| IBIS file MPC8308_ibis.ibs generated by Viper version: 2008.08.r27
[IBIS Ver]   4.2
[Comment Char]   |_char
[File Name]   mpc8308_ibis_19072011.ibs
[File Rev]   B
[Date]   Mon Nov 2 12:15:30 2009
[Source]   Generated using: Viper
[Notes]   Updated pulldown data  for ddr1_type_drv_io model.
[Disclaimer]
[Copyright]   Copyright (C) 1998 - 2004 Freescale Semiconductor Israel Ltd.
|   MPC8308
[Component]   MPC8308
[Manufacturer]   FREESCALE
[Package]
| variable   typ   min   max
R_pkg   326.285m   89.855m   584.065m
L_pkg   4.52nH   1.32nH   7.74nH
C_pkg   1.88pF   0.974pF   6.09pF
[Pin] signal_name   model_name   R_pin   L_pin   C_pin
A1   GVDD   POWER   2.35E-01  3.44E-09  4.55E-12
A10   XPADVSS   GND   NA   NA   NA
A11   SD_IMP_CAL_TX   tx_pzctl   4.46E-01  5.33E-09  9.95E-13
A12   XCOREVSS   GND   NA   NA   NA
A13   RXA   ptrmr100_cm   4.10E-01  4.92E-09  1.01E-12
A14   XCOREVDD   POWER   1.42E-01  2.40E-09  3.60E-12
A15   SD_IMP_CAL_RX   rx_pzctl   5.04E-01  6.02E-09  1.03E-12
A16   NVDDB   POWER   3.74E-01  5.65E-09  2.94E-12
A17   IRQ_B0   Progbuffer1   4.01E-01  5.91E-09  1.08E-12
A18   IRQ_B3   Progbuffer1   4.06E-01  5.79E-09  1.14E-12
A19   NVDDB   POWER   3.74E-01  5.65E-09  2.94E-12
A2   VSS   GND   NA   NA   NA
A20   TSEC1_MDC   Progbuffer1   4.23E-01  6.17E-09  1.26E-12
A21   VSS   GND   NA   NA   NA
A22   TSEC1_RX_CLK   Progbuffer1   3.77E-01  6.03E-09  1.75E-12
A23   NVDDC   POWER   4.46E-01  5.97E-09  4.02E-12
A3   MEMC_MCK0   Progbuffer2   4.19E-01  6.14E-09  1.33E-12
A4   MEMC_MCK_B0   Progbuffer2   4.10E-01  6.18E-09  1.30E-12
A5   MEMC_MODT0   Progbuffer2   4.18E-01  6.07E-09  1.18E-12
A6   GVDD   POWER   2.35E-01  3.44E-09  4.55E-12
A7   SD_CD_B   Progbuffer1   3.90E-01  5.44E-09  1.24E-12
A8   SD_DAT2   Progbuffer1   3.81E-01  5.40E-09  1.20E-12
A9   IIC_SCL1   Progbuffer1   4.00E-01  5.74E-09  1.05E-12
AA1   MEMC_MDQ5   Progbuffer2   4.30E-01  6.08E-09  1.53E-12
AA10  LGPL1   Progbuffer1   3.51E-01  4.78E-09  1.18E-12
AA11  NVDDK   POWER   1.50E-01  2.43E-09  6.05E-12
AA12  LCS_B2   Progbuffer1   3.61E-01  4.89E-09  1.29E-12
AA13  LCS_B0   Progbuffer1   3.61E-01  4.88E-09  1.29E-12
AA14  LA20   Progbuffer1   3.52E-01  4.95E-09  1.32E-12
AA15  LA12   Progbuffer1   3.58E-01  4.62E-09  1.34E-12
AA16  LA7   Progbuffer1   3.62E-01  5.03E-09  1.48E-12
AA17  LA5   Progbuffer1   3.75E-01  5.29E-09  1.43E-12
AA18  LA4   Progbuffer1   3.88E-01  5.52E-09  1.46E-12
AA19  LD14   Progbuffer1   3.96E-01  5.64E-09  1.52E-12
AA2   MEMC_MDQ4   Progbuffer2   4.01E-01  5.83E-09  1.64E-12
AA20  LD9   Progbuffer1   4.03E-01  5.73E-09  1.47E-12
AA21  LD4   Progbuffer1   4.06E-01  5.85E-09  1.62E-12
AA22  STBY_VBAT   POWER   2.25E-01  3.87E-09  1.83E-12
AA23  RTC_PIT_CLOCK   Progbuffer1   4.29E-01  6.45E-09  1.34E-12
AA3   MEMC_MDQ3   Progbuffer2   3.92E-01  5.55E-09  1.55E-12
AA4   VSS   GND   NA   NA   NA
AA5   SPICLK   Progbuffer1   3.43E-01  4.74E-09  1.42E-12
AA6   TMS   Progbuffer1   3.67E-01  5.05E-09  1.34E-12
AA7   QUIESCE_B   Progbuffer1   3.63E-01  4.98E-09  1.27E-12
AA8   PORESET_B   Progbuffer1   3.50E-01  4.77E-09  1.23E-12
AA9   HRESET_B   Progbuffer1   3.53E-01  4.75E-09  1.26E-12
AB1   VSS   GND   NA   NA   NA
AB10  LGPL2   Progbuffer1   3.80E-01  4.89E-09  1.17E-12
AB11  LWE_B0   Progbuffer1   3.46E-01  4.72E-09  1.20E-12
AB12  VSS   GND   NA   NA   NA
AB13  LCS_B1   Progbuffer1   3.82E-01  5.40E-09  1.38E-12
AB14  LA21   Progbuffer1   3.71E-01  5.30E-09  1.27E-12
AB15  LA19   Progbuffer1   3.80E-01  5.48E-09  1.33E-12
AB16  NVDDK   POWER   1.50E-01  2.43E-09  6.05E-12
AB17  LA11   Progbuffer1   3.92E-01  5.66E-09  1.37E-12
AB18  LA8   Progbuffer1   4.06E-01  5.89E-09  1.49E-12
AB19  VSS   GND   NA   NA   NA
AB2   MEMC_MDM0   Progbuffer2   4.21E-01  6.20E-09  1.52E-12
AB20  LD12   Progbuffer1   4.21E-01  6.12E-09  1.50E-12
AB21  LD7   Progbuffer1   4.37E-01  6.14E-09  1.54E-12
AB22  NVDDK   POWER   1.50E-01  2.43E-09  6.05E-12
AB23  NVDDJ   POWER   3.92E-01  5.82E-09  1.51E-12
AB3   MEMC_MDQ2   Progbuffer2   3.99E-01  5.92E-09  1.57E-12
AB4   SPISEL   Progbuffer1   3.73E-01  5.49E-09  1.44E-12
AB5   SPIMOSI   Progbuffer1   3.84E-01  5.45E-09  1.34E-12
AB6   VSS   GND   NA   NA   NA
AB7   SRESET_B   Progbuffer1   3.87E-01  5.24E-09  1.25E-12
AB8   NVDDP   POWER   1.50E-01  2.43E-09  6.05E-12
AB9   LGPL4   Progbuffer1   3.69E-01  5.11E-09  1.22E-12
AC1   GVDD   POWER   2.35E-01  3.44E-09  4.55E-12
AC10  LGPL3   Progbuffer1   3.90E-01  5.49E-09  1.04E-12
AC11  LWE_B1   Progbuffer1   3.70E-01  5.17E-09  1.22E-12
AC12  LCLK0   Progbuffer1   3.22E-01  4.34E-09  1.35E-12
AC13  NVDDK   POWER   1.50E-01  2.43E-09  6.05E-12
AC14  LA25   Progbuffer1   4.15E-01  5.88E-09  1.18E-12
AC15  LA15   Progbuffer1   3.91E-01  5.37E-09  1.22E-12
AC16  LA13   Progbuffer1   4.12E-01  5.89E-09  1.18E-12
AC17  LD15   Progbuffer1   3.90E-01  5.61E-09  1.46E-12
AC18  LA9   Progbuffer1   4.29E-01  6.14E-09  1.25E-12
AC19  LA6   Progbuffer1   4.31E-01  6.45E-09  1.27E-12
AC2   VSS   GND   NA   NA   NA
AC20  LA0   Progbuffer1   4.38E-01  6.54E-09  1.31E-12
AC21  LD11   Progbuffer1   4.44E-01  6.62E-09  1.33E-12
AC22  LD5   Progbuffer1   4.50E-01  6.71E-09  1.37E-12
AC23  VSS   GND   NA   NA   NA
AC3   MEMC_MDQS0   Progbuffer2   3.56E-01  5.44E-09  1.71E-12
AC4   NVDDP   POWER   1.50E-01  2.43E-09  6.05E-12
AC5   TDO   Progbuffer1   4.17E-01  5.78E-09  1.15E-12
AC6   TEST_MODE   Progbuffer1   3.98E-01  5.75E-09  1.42E-12
AC7   THERM0   Progbuffer1   3.98E-01  5.69E-09  1.11E-12
AC8   SYS_CLK_IN   Progbuffer1   3.33E-01  4.31E-09  1.32E-12
AC9   VSS   GND   NA   NA   NA
B1   VSS   GND   NA   NA   NA
B10   NVDDA   POWER   5.84E-01  7.74E-09  2.08E-12
B12   XCOREVDD   POWER   1.42E-01  2.40E-09  3.60E-12
B13   RXA_B   ptrmr100_cm   4.19E-01  5.41E-09  9.74E-13
B14   XCOREVSS   GND   NA   NA   NA
B15   XPADVSS   GND   NA   NA   NA
B17   IRQ_B2   Progbuffer1   3.79E-01  5.27E-09  1.28E-12
B18   UART_SIN1   Progbuffer1   3.86E-01  5.42E-09  1.29E-12
B19   VSS   GND   NA   NA   NA
B2   MEMC_MBA1   Progbuffer2   4.31E-01  6.26E-09  1.61E-12
B20   TSEC1_COL   Progbuffer1   4.00E-01  5.55E-09  1.44E-12
B21   TSEC1_CRS   Progbuffer1   4.09E-01  6.01E-09  1.66E-12
B22   NVDDC   POWER   4.46E-01  5.97E-09  4.02E-12
B23   VSS   GND   NA   NA   NA
B3   GVDD   POWER   2.35E-01  3.44E-09  4.55E-12
B4   MEMC_MRAS_B   Progbuffer2   4.12E-01  5.84E-09  1.29E-12
B5   MEMC_MODT1   Progbuffer2   3.96E-01  5.64E-09  1.36E-12
B6   MEMC_MCS_B0   Progbuffer2   3.95E-01  5.51E-09  1.29E-12
B7   NVDDA   POWER   5.84E-01  7.74E-09  2.08E-12
B8   SD_DAT1   Progbuffer1   3.54E-01  4.87E-09  1.23E-12
B9   SD_DAT3   Progbuffer1   3.76E-01  5.12E-09  1.23E-12
C1   MEMC_MA10   Progbuffer2   4.47E-01  6.37E-09  1.34E-12
C10   IIC_SCL2   Progbuffer1   3.68E-01  4.89E-09  1.03E-12
C11   XCOREVSS   GND   NA   NA   NA
C12   SD_REF_CLK_B   ptrmr100_cm   3.86E-01  3.95E-09  1.24E-12
C13   XCOREVDD   POWER   1.42E-01  2.40E-09  3.60E-12
C14   TXA   tx_select   3.56E-01  4.78E-09  1.04E-12
C15   TXA_B   tx_select   3.89E-01  4.01E-09  1.07E-12
C16   VSS   GND   NA   NA   NA
C17   UART_SOUT1   Progbuffer1   3.63E-01  4.99E-09  1.33E-12
C18   NVDDB   POWER   3.74E-01  5.65E-09  2.94E-12
C19   TSEC1_MDIO   Progbuffer1   3.76E-01  5.23E-09  1.38E-12
C2   MEMC_MA0   Progbuffer2   4.29E-01  5.96E-09  1.61E-12
C20   TSEC1_RXD1   Progbuffer1   3.87E-01  5.59E-09  1.64E-12
C21   TSEC1_RXD2   Progbuffer1   3.90E-01  5.55E-09  1.46E-12
C22   TSEC1_RXD3   Progbuffer1   4.07E-01  5.90E-09  1.43E-12
C23   TSEC1_RX_ER   Progbuffer1   4.23E-01  6.20E-09  1.29E-12
C3   MEMC_MBA0   Progbuffer2   4.01E-01  5.71E-09  1.56E-12
C4   VSS   GND   NA   NA   NA
C5   MEMC_MCAS_B   Progbuffer2   3.68E-01  5.10E-09  1.38E-12
C6   MEMC_MCS_B1   Progbuffer2   3.77E-01  4.73E-09  1.31E-12
C7   NVDDA   POWER   5.84E-01  7.74E-09  2.08E-12
C8   SD_DAT0   Progbuffer1   3.50E-01  4.30E-09  1.21E-12
C9   IIC_SDA1   Progbuffer1   3.34E-01  4.26E-09  1.26E-12
D1   GVDD   POWER   2.35E-01  3.44E-09  4.55E-12
D10   IIC_SDA2   Progbuffer1   2.93E-01  3.86E-09  1.41E-12
D11   XCOREVSS   GND   NA   NA   NA
D12   SD_REF_CLK   ptrmr100_cm   3.46E-01  4.30E-09  1.23E-12
D13   XCOREVSS   GND   NA   NA   NA
D14   XPADVSS   GND   NA   NA   NA
D15   XPADVDD   POWER   2.04E-01  2.96E-09  2.44E-12
D17   UART_SOUT2   Progbuffer1   3.57E-01  4.45E-09  1.34E-12
D18   UART_SIN2   Progbuffer1   3.57E-01  4.77E-09  1.37E-12
D19   VSS   GND   NA   NA   NA
D2   MEMC_MA1   Progbuffer2   4.13E-01  5.94E-09  1.47E-12
D20   TSEC1_RXD0   Progbuffer1   3.63E-01  5.08E-09  1.53E-12
D21   TSEC1_RX_DV   Progbuffer1   3.82E-01  5.44E-09  1.42E-12
D22   TSEC1_TXD0   Progbuffer1   4.01E-01  5.76E-09  1.39E-12
D23   NVDDC   POWER   4.46E-01  5.97E-09  4.02E-12
D3   MEMC_MA2   Progbuffer2   4.15E-01  5.34E-09  1.54E-12
D4   MEMC_MA3   Progbuffer2   3.66E-01  5.13E-09  1.56E-12
D5   MEMC_MWE_B   Progbuffer2   3.76E-01  4.73E-09  1.54E-12
D6   VSS   GND   NA   NA   NA
D7   SD_CLK   Progbuffer1   3.49E-01  4.40E-09  1.14E-12
D8   SD_WP   Progbuffer1   3.31E-01  4.41E-09  1.40E-12
D9   NVDDA   POWER   5.84E-01  7.74E-09  2.08E-12
E1   MEMC_MA7   Progbuffer2   4.18E-01  6.10E-09  1.20E-12
E2   MEMC_MA6   Progbuffer2   3.99E-01  5.66E-09  1.38E-12
E20   NVDDC   POWER   4.46E-01  5.97E-09  4.02E-12
E21   TSEC1_TXD1   Progbuffer1   3.76E-01  5.28E-09  1.33E-12
E22   TSEC1_TX_ER   Progbuffer1   3.94E-01  5.60E-09  1.35E-12
E23   TSEC1_TX_CLK   Progbuffer1   3.45E-01  4.53E-09  1.55E-12
E3   VSS   GND   NA   NA   NA
E4   MEMC_MA4   Progbuffer2   3.67E-01  5.06E-09  1.48E-12
F1   GVDD   POWER   2.35E-01  3.44E-09  4.55E-12
F10   XPADVDD   POWER   2.04E-01  2.96E-09  2.44E-12
F11   SD_PLL_TPA_ANA   pad_ae   3.68E-01  3.88E-09  1.30E-12
F12   SDAVSS_0   GND   NA   NA   NA
F13   SD_PLL_TPD   pouv_out   3.43E-01  4.45E-09  1.40E-12
F14   XPADVDD   POWER   2.04E-01  2.96E-09  2.44E-12
F15   VSS   GND   NA   NA   NA
F16   IRQ_B1   Progbuffer1   3.44E-01  4.62E-09  1.46E-12
F17   VSS   GND   NA   NA   NA
F18   TSEC1_GTX_CLK   Progbuffer1   2.67E-01  3.07E-09  1.52E-12
F2   MEMC_MA8   Progbuffer2   3.90E-01  5.56E-09  1.40E-12
F20   TSEC1_TX_EN   Progbuffer1   3.51E-01  4.76E-09  1.34E-12
F21   TSEC1_TXD2   Progbuffer1   3.75E-01  5.23E-09  1.32E-12
F22   TSEC1_TXD3   Progbuffer1   3.90E-01  5.49E-09  1.33E-12
F23   VSS   GND   NA   NA   NA
F3   MEMC_MA9   Progbuffer2   3.75E-01  5.12E-09  1.37E-12
F4   MEMC_MA5   Progbuffer2   3.56E-01  4.86E-09  1.39E-12
F6   GVDD   POWER   2.35E-01  3.44E-09  4.55E-12
F7   MEMC_MA11   Progbuffer2   3.28E-01  4.28E-09  1.43E-12
F8   VSS   GND   NA   NA   NA
F9   NVDDA   POWER   5.84E-01  7.74E-09  2.08E-12
G1   MEMC_MCK2   Progbuffer2   3.89E-01  5.64E-09  1.21E-12
G10   VSS   GND   NA   NA   NA
G11   XCOREVSS   GND   NA   NA   NA
G12   SDAVDD_0   POWER   3.65E-01  4.85E-09  1.49E-12
G13   XPADVSS   GND   NA   NA   NA
G14   XPADVSS   GND   NA   NA   NA
G15   VSS   GND   NA   NA   NA
G16   VSS   GND   NA   NA   NA
G17   VSS   GND   NA   NA   NA
G18   NVDDC   POWER   4.46E-01  5.97E-09  4.02E-12
G2   MEMC_MA12   Progbuffer2   3.87E-01  5.48E-09  1.39E-12
G20   VSS   GND   NA   NA   NA
G21   GPIO_0   Progbuffer1   3.65E-01  5.05E-09  1.27E-12
G22   NVDDF   POWER   2.32E-01  3.22E-09  3.90E-12
G23   GPIO_3   Progbuffer1   3.47E-01  4.68E-09  1.22E-12
G3   MEMC_MA13   Progbuffer2   3.69E-01  5.12E-09  1.42E-12
G4   GVDD   POWER   2.35E-01  3.44E-09  4.55E-12
G6   MEMC_MVREF   Progbuffer2   1.31E-01  1.93E-09  1.74E-12
G7   VSS   GND   NA   NA   NA
G8   VSS   GND   NA   NA   NA
G9   SD_CMD   Progbuffer1   3.55E-01  4.81E-09  1.52E-12
H1   MEMC_MCK_B2   Progbuffer2   3.89E-01  5.72E-09  1.18E-12
H10   VDD   POWER   8.99E-02  1.32E-09  2.08E-12
H11   XCOREVSS   GND   NA   NA   NA
H12   XPADVSS   GND   NA   NA   NA
H13   XCOREVSS   GND   NA   NA   NA
H14   VDD   POWER   8.99E-02  1.32E-09  2.08E-12
H15   VDD   POWER   8.99E-02  1.32E-09  2.08E-12
H16   VDD   POWER   8.99E-02  1.32E-09  2.08E-12
H17   VSS   GND   NA   NA   NA
H18   GPIO_2   Progbuffer1   2.38E-01  2.74E-09  1.52E-12
H2   VSS   GND   NA   NA   NA
H20   GPIO_8   Progbuffer1   3.39E-01  4.55E-09  1.29E-12
H21   GPIO_7   Progbuffer1   3.59E-01  4.93E-09  1.30E-12
H22   GPIO_6   Progbuffer1   3.74E-01  5.21E-09  1.26E-12
H23   VSS   GND   NA   NA   NA
H3   MEMC_MCKE   Progbuffer2   3.38E-01  4.53E-09  1.24E-12
H4   MEMC_MBA2   Progbuffer2   3.32E-01  4.37E-09  1.56E-12
H6   VSS   GND   NA   NA   NA
H7   VSS   GND   NA   NA   NA
H8   VDD   POWER   8.99E-02  1.32E-09  2.08E-12
H9   VDD   POWER   8.99E-02  1.32E-09  2.08E-12
J1   GVDD   POWER   2.35E-01  3.44E-09  4.55E-12
J10   VSS   GND   NA   NA   NA
J11   VSS   GND   NA   NA   NA
J12   VSS   GND   NA   NA   NA
J13   VSS   GND   NA   NA   NA
J14   VSS   GND   NA   NA   NA
J15   VSS   GND   NA   NA   NA
J16   VDD   POWER   8.99E-02  1.32E-09  2.08E-12
J17   GPIO_14   Progbuffer1   3.60E-01  4.91E-09  1.59E-12
J18   GPIO_4   Progbuffer1   3.36E-01  4.48E-09  1.35E-12
J2   MEMC_MECC4   Progbuffer2   3.71E-01  5.16E-09  1.26E-12
J20   GPIO_5   Progbuffer1   3.34E-01  4.50E-09  1.23E-12
J21   GPIO_9   Progbuffer1   3.53E-01  4.85E-09  1.25E-12
J22   NVDDF   POWER   2.32E-01  3.22E-09  3.90E-12
J23   GPIO_10   Progbuffer1   3.40E-01  4.46E-09  1.13E-12
J3   MEMC_MECC6   Progbuffer2   3.57E-01  4.87E-09  1.27E-12
J4   GVDD   POWER   2.35E-01  3.44E-09  4.55E-12
J6   MEMC_MECC7   Progbuffer2   3.41E-01  4.39E-09  1.32E-12
J7   VSS   GND   NA   NA   NA
J8   VDD   POWER   8.99E-02  1.32E-09  2.08E-12
J9   VSS   GND   NA   NA   NA
K1   MEMC_MDQS8   Progbuffer2   2.94E-01  3.77E-09  1.54E-12
K10   VSS   GND   NA   NA   NA
K11   VSS   GND   NA   NA   NA
K12   VSS   GND   NA   NA   NA
K13   VSS   GND   NA   NA   NA
K14   VSS   GND   NA   NA   NA
K15   VSS   GND   NA   NA   NA
K16   VDD   POWER   8.99E-02  1.32E-09  2.08E-12
K17   NVDDF   POWER   2.32E-01  3.22E-09  3.90E-12
K18   GPIO_13   Progbuffer1   3.29E-01  4.38E-09  1.34E-12
K2   MEMC_MDM8   Progbuffer2   3.69E-01  5.17E-09  1.25E-12
K20   GPIO_12   Progbuffer1   3.26E-01  4.36E-09  1.20E-12
K21   GPIO_15   Progbuffer1   3.47E-01  4.77E-09  1.20E-12
K22   GPIO_11   Progbuffer1   3.70E-01  5.15E-09  1.22E-12
K23   GPIO_1   Progbuffer1   3.92E-01  5.51E-09  1.05E-12
K3   MEMC_MECC3   Progbuffer2   3.46E-01  4.76E-09  1.22E-12
K4   MEMC_MECC2   Progbuffer2   3.27E-01  4.39E-09  1.21E-12
K6   MEMC_MECC5   Progbuffer2   3.39E-01  4.54E-09  1.34E-12
K7   GVDD   POWER   2.35E-01  3.44E-09  4.55E-12
K8   VDD   POWER   8.99E-02  1.32E-09  2.08E-12
K9   VSS   GND   NA   NA   NA
L1   VSS   GND   NA   NA   NA
L10   VSS   GND   NA   NA   NA
L11   VSS   GND   NA   NA   NA
L12   VSS   GND   NA   NA   NA
L13   VSS   GND   NA   NA   NA
L14   VSS   GND   NA   NA   NA
L15   VSS   GND   NA   NA   NA
L16   VDD   POWER   8.99E-02  1.32E-09  2.08E-12
L17   TSEC_TMR_GCLK   Progbuffer1   3.43E-01  4.63E-09  1.75E-12
L18   TSEC_TMR_PP1   Progbuffer1   3.42E-01  4.69E-09  1.35E-12
L2   MEMC_MDQ30   Progbuffer2   3.59E-01  5.01E-09  1.22E-12
L20   VSS   GND   NA   NA   NA
L21   TSEC_TMR_PP2   Progbuffer1   3.41E-01  4.72E-09  1.18E-12
L22   TSEC_TMR_PP3   Progbuffer1   3.66E-01  5.11E-09  1.20E-12
L23   TSEC_TMR_ALARM1   Progbuffer1   3.81E-01  5.53E-09  1.05E-12
L3   MEMC_MDQ31   Progbuffer2   3.39E-01  4.63E-09  1.23E-12
L4   MEMC_MECC0   Progbuffer2   3.23E-01  4.32E-09  1.24E-12
L6   MEMC_MECC1   Progbuffer2   3.37E-01  4.37E-09  1.30E-12
L7   VSS   GND   NA   NA   NA
L8   VDD   POWER   8.99E-02  1.32E-09  2.08E-12
L9   VSS   GND   NA   NA   NA
M1   MEMC_MDQS3   Progbuffer2   2.87E-01  3.91E-09  1.44E-12
M10   VSS   GND   NA   NA   NA
M11   VSS   GND   NA   NA   NA
M12   VSS   GND   NA   NA   NA
M13   VSS   GND   NA   NA   NA
M14   VSS   GND   NA   NA   NA
M15   VSS   GND   NA   NA   NA
M16   VDD   POWER   8.99E-02  1.32E-09  2.08E-12
M17   NVDDG   POWER   1.49E-01  1.84E-09  6.09E-12
M18   TSEC1_TMR_RX_ESFD   Progbuffer1   3.21E-01  4.28E-09  1.39E-12
M2   MEMC_MDQ28   Progbuffer2   3.59E-01  5.00E-09  1.22E-12
M20   TSEC1_TMR_TX_ESFD   Progbuffer1   3.19E-01  4.24E-09  1.22E-12
M21   TSEC2_CRS   Progbuffer1   3.40E-01  4.72E-09  1.27E-12
M22   GPIO_7A   Progbuffer1   3.60E-01  5.08E-09  1.22E-12
M23   TSEC_TMR_ALARM2   Progbuffer1   3.85E-01  5.49E-09  1.06E-12
M3   MEMC_MDQ29   Progbuffer2   3.43E-01  4.61E-09  1.25E-12
M4   VSS   GND   NA   NA   NA
M6   MEMC_MDQ27   Progbuffer2   3.24E-01  4.38E-09  1.30E-12
M7   MEMC_MDM3   Progbuffer2   3.31E-01  4.54E-09  1.46E-12
M8   VDD   POWER   8.99E-02  1.32E-09  2.08E-12
M9   VSS   GND   NA   NA   NA
N1   GVDD   POWER   2.35E-01  3.44E-09  4.55E-12
N10   VSS   GND   NA   NA   NA
N11   VSS   GND   NA   NA   NA
N12   VSS   GND   NA   NA   NA
N13   VSS   GND   NA   NA   NA
N14   VSS   GND   NA   NA   NA
N15   VSS   GND   NA   NA   NA
N16   VDD   POWER   8.99E-02  1.32E-09  2.08E-12
N17   GPIO_5A   Progbuffer1   3.40E-01  4.61E-09  1.58E-12
N18   GTM1_TIN4   Progbuffer1   3.24E-01  4.34E-09  1.39E-12
N2   MEMC_MDQ26   Progbuffer2   3.59E-01  5.07E-09  1.20E-12
N20   GTM1_TGATE3_B   Progbuffer1   3.20E-01  4.34E-09  1.21E-12
N21   TSEC0_TMR_TX_ESFD   Progbuffer1   3.38E-01  4.67E-09  1.23E-12
N22   NVDDG   POWER   1.49E-01  1.84E-09  6.09E-12
N23   TSEC0_TMR_RX_ESFD   Progbuffer1   3.86E-01  5.38E-09  1.03E-12
N3   MEMC_MDQ25   Progbuffer2   3.37E-01  4.64E-09  1.24E-12
N4   MEMC_MDQ24   Progbuffer2   3.19E-01  4.26E-09  1.24E-12
N6   MEMC_MDQ21   Progbuffer2   3.13E-01  4.14E-09  1.38E-12
N7   GVDD   POWER   2.35E-01  3.44E-09  4.55E-12
N8   VDD   POWER   8.99E-02  1.32E-09  2.08E-12
N9   VSS   GND   NA   NA   NA
P1   MEMC_MDQ23   Progbuffer2   3.79E-01  5.42E-09  1.06E-12
P10   VSS   GND   NA   NA   NA
P11   VSS   GND   NA   NA   NA
P12   VSS   GND   NA   NA   NA
P13   VSS   GND   NA   NA   NA
P14   VSS   GND   NA   NA   NA
P15   VSS   GND   NA   NA   NA
P16   VDD   POWER   8.99E-02  1.32E-09  2.08E-12
P17   NVDDH   POWER   2.46E-01  3.33E-09  4.23E-12
P18   USBDR_NXT   Progbuffer1   3.40E-01  4.46E-09  1.33E-12
P2   MEMC_MDQ22   Progbuffer2   3.66E-01  4.88E-09  1.23E-12
P20   USBDR_PWRFAULT   Progbuffer1   3.27E-01  4.41E-09  1.22E-12
P21   GPIO_6A   Progbuffer1   3.44E-01  4.73E-09  1.19E-12
P22   GTM1_TIN3   Progbuffer1   3.62E-01  5.06E-09  1.21E-12
P23   GTM1_TGATE4_B   Progbuffer1   3.87E-01  5.49E-09  1.08E-12
P3   MEMC_MDM2   Progbuffer2   3.41E-01  4.68E-09  1.22E-12
P4   MEMC_MDQ20   Progbuffer2   3.22E-01  4.32E-09  1.24E-12
P6   VSS   GND   NA   NA   NA
P7   VSS   GND   NA   NA   NA
P8   VDD   POWER   8.99E-02  1.32E-09  2.08E-12
P9   VSS   GND   NA   NA   NA
R1   MEMC_MDQS2   Progbuffer2   3.02E-01  4.02E-09  1.36E-12
R10   VSS   GND   NA   NA   NA
R11   VSS   GND   NA   NA   NA
R12   VSS   GND   NA   NA   NA
R13   VSS   GND   NA   NA   NA
R14   VSS   GND   NA   NA   NA
R15   VSS   GND   NA   NA   NA
R16   VDD   POWER   8.99E-02  1.32E-09  2.08E-12
R17   USBDR_PCTL0   Progbuffer1   3.61E-01  4.85E-09  1.54E-12
R18   USBDR_TXDRXD5   Progbuffer1   3.35E-01  4.48E-09  1.36E-12
R2   VSS   GND   NA   NA   NA
R20   NVDDH   POWER   2.46E-01  3.33E-09  4.23E-12
R21   USBDR_DIR   Progbuffer1   3.59E-01  4.70E-09  1.25E-12
R22   VSS   GND   NA   NA   NA
R23   USBDR_CLK   Progbuffer1   3.95E-01  5.64E-09  1.07E-12
R3   MEMC_MDQ19   Progbuffer2   3.49E-01  4.74E-09  1.23E-12
R4   MEMC_MDQ18   Progbuffer2   3.41E-01  4.70E-09  1.44E-12
R6   AVDD1   POWER   1.45E-01  1.84E-09  1.53E-12
R7   VSS   GND   NA   NA   NA
R8   VDD   POWER   8.99E-02  1.32E-09  2.08E-12
R9   VSS   GND   NA   NA   NA
T1   GVDD   POWER   2.35E-01  3.44E-09  4.55E-12
T10   VDD   POWER   8.99E-02  1.32E-09  2.08E-12
T11   VDD   POWER   8.99E-02  1.32E-09  2.08E-12
T12   VDD   POWER   8.99E-02  1.32E-09  2.08E-12
T13   VDD   POWER   8.99E-02  1.32E-09  2.08E-12
T14   VDD   POWER   8.99E-02  1.32E-09  2.08E-12
T15   VDD   POWER   8.99E-02  1.32E-09  2.08E-12
T16   VDD   POWER   8.99E-02  1.32E-09  2.08E-12
T17   NVDDH   POWER   2.46E-01  3.33E-09  4.23E-12
T18   GTM1_TOUT3_B   Progbuffer1   3.29E-01  4.36E-09  1.34E-12
T2   MEMC_MDQ17   Progbuffer2   3.72E-01  5.19E-09  1.24E-12
T20   USBDR_TXDRXD4   Progbuffer1   3.51E-01  4.50E-09  1.32E-12
T21   USBDR_TXDRXD1   Progbuffer1   3.61E-01  4.95E-09  1.27E-12
T22   USBDR_TXDRXD0   Progbuffer1   3.82E-01  5.24E-09  1.26E-12
T23   NVDDH   POWER   2.46E-01  3.33E-09  4.23E-12
T3   MEMC_MDQ16   Progbuffer2   3.57E-01  4.91E-09  1.26E-12
T4   GVDD   POWER   2.35E-01  3.44E-09  4.55E-12
T6   VSS   GND   NA   NA   NA
T7   VSS   GND   NA   NA   NA
T8   VDD   POWER   8.99E-02  1.32E-09  2.08E-12
T9   VDD   POWER   8.99E-02  1.32E-09  2.08E-12
U1   MEMC_MCK_B1   Progbuffer2   3.74E-01  5.36E-09  1.42E-12
U10   NVDDK   POWER   1.50E-01  2.43E-09  6.05E-12
U11   LBCTL   Progbuffer1   3.61E-01  5.02E-09  1.75E-12
U12   LA22   Progbuffer1   3.39E-01  4.70E-09  1.73E-12
U13   LA16   Progbuffer1   3.47E-01  4.79E-09  1.67E-12
U14   NVDDK   POWER   1.50E-01  2.43E-09  6.05E-12
U15   LA2   Progbuffer1   3.65E-01  4.93E-09  1.65E-12
U16   LD2   Progbuffer1   3.57E-01  4.55E-09  1.71E-12
U17   VSS   GND   NA   NA   NA
U18   LD0   Progbuffer1   3.22E-01  4.49E-09  1.84E-12
U2   MEMC_MCK1   Progbuffer2   3.77E-01  5.40E-09  1.41E-12
U20   USBDR_PCTL1   Progbuffer1   3.48E-01  4.72E-09  1.37E-12
U21   VSS   GND   NA   NA   NA
U22   USBDR_TXDRXD3   Progbuffer1   3.91E-01  5.44E-09  1.31E-12
U23   USBDR_TXDRXD2   Progbuffer1   4.08E-01  5.96E-09  1.15E-12
U3   MEMC_MDQ13   Progbuffer2   3.63E-01  5.03E-09  1.29E-12
U4   MEMC_MDQ12   Progbuffer2   3.59E-01  4.59E-09  1.39E-12
U6   MEMC_MDQ15   Progbuffer2   3.20E-01  4.23E-09  1.59E-12
U7   GVDD   POWER   2.35E-01  3.44E-09  4.55E-12
U8   VSS   GND   NA   NA   NA
U9   TDI   Progbuffer1   3.55E-01  4.75E-09  1.54E-12
V1   MEMC_MDQS1   Progbuffer2   3.61E-01  4.59E-09  1.68E-12
V10   AVDD2   POWER   2.22E-01  2.67E-09  1.30E-12
V11   VSS   GND   NA   NA   NA
V12   LA23   Progbuffer1   3.33E-01  4.35E-09  1.53E-12
V13   LA17   Progbuffer1   3.16E-01  4.28E-09  1.54E-12
V14   LA10   Progbuffer1   3.30E-01  4.44E-09  1.41E-12
V15   LA3   Progbuffer1   3.38E-01  4.56E-09  1.40E-12
V16   LD13   Progbuffer1   3.41E-01  4.32E-09  1.37E-12
V17   LD6   Progbuffer1   3.38E-01  4.59E-09  1.45E-12
V18   LD1   Progbuffer1   3.15E-01  4.19E-09  1.40E-12
V2   VSS   GND   NA   NA   NA
V20   GTM1_TOUT4_B   Progbuffer1   3.30E-01  4.38E-09  1.38E-12
V21   USBDR_STP   Progbuffer1   3.75E-01  5.17E-09  1.33E-12
V22   USBDR_TXDRXD7   Progbuffer1   3.94E-01  5.62E-09  1.34E-12
V23   USBDR_TXDRXD6   Progbuffer1   4.14E-01  6.02E-09  1.13E-12
V3   MEMC_MDM1   Progbuffer2   3.77E-01  5.27E-09  1.38E-12
V4   MEMC_MDQ14   Progbuffer2   3.59E-01  5.02E-09  1.49E-12
V6   MEMC_MDQ0   Progbuffer2   2.95E-01  4.04E-09  1.65E-12
V7   VSS   GND   NA   NA   NA
V8   TRST_B   Progbuffer1   3.24E-01  4.27E-09  1.48E-12
V9   VSS   GND   NA   NA   NA
W1   MEMC_MDQ9   Progbuffer2   4.33E-01  6.42E-09  1.27E-12
W2   MEMC_MDQ11   Progbuffer2   4.03E-01  5.74E-09  1.40E-12
W20   VSS   GND   NA   NA   NA
W21   TSEC_TMR_TRIG1   Progbuffer1   3.67E-01  4.92E-09  1.38E-12
W22   NVDDH   POWER   2.46E-01  3.33E-09  4.23E-12
W23   TSEC_TMR_CLK   Progbuffer1   4.20E-01  6.17E-09  1.23E-12
W3   MEMC_MDQ8   Progbuffer2   3.98E-01  5.41E-09  1.49E-12
W4   MEMC_MDQ6   Progbuffer2   3.67E-01  5.19E-09  1.57E-12
Y1   MEMC_MDQ10   Progbuffer2   4.22E-01  5.74E-09  1.49E-12
Y10   LGPL0   Progbuffer1   3.35E-01  4.30E-09  1.14E-12
Y11   LCS_B3   Progbuffer1   3.29E-01  4.08E-09  1.32E-12
Y12   LA24   Progbuffer1   3.16E-01  4.23E-09  1.17E-12
Y13   LA18   Progbuffer1   3.19E-01  4.14E-09  1.14E-12
Y14   LA14   Progbuffer1   3.18E-01  4.22E-09  1.79E-12
Y15   VSS   GND   NA   NA   NA
Y16   LA1   Progbuffer1   3.37E-01  4.54E-09  1.39E-12
Y17   LD10   Progbuffer1   3.30E-01  4.46E-09  1.52E-12
Y18   NVDDK   POWER   1.50E-01  2.43E-09  6.05E-12
Y19   LD8   Progbuffer1   3.73E-01  5.21E-09  1.50E-12
Y2   MEMC_MDQ7   Progbuffer2   4.10E-01  6.00E-09  1.54E-12
Y20   LD3   Progbuffer1   3.81E-01  5.34E-09  1.53E-12
Y21   TSEC_TMR_TRIG2   Progbuffer1   3.92E-01  5.38E-09  1.46E-12
Y22   STBY_BYPASS   Progbuffer1   3.95E-01  5.77E-09  1.48E-12
Y23   STBY_1V   POWER   3.01E-01  4.51E-09  1.57E-12
Y3   GVDD   POWER   2.35E-01  3.44E-09  4.55E-12
Y4   MEMC_MDQ1   Progbuffer2   3.20E-01  4.44E-09  1.68E-12
Y5   NVDDP   POWER   1.50E-01  2.43E-09  6.05E-12
Y6   SPIMISO   Progbuffer1   3.10E-01  4.18E-09  1.37E-12
Y7   TCK   Progbuffer1   3.41E-01  4.59E-09  1.25E-12
Y8   VSS   GND   NA   NA   NA
Y9   LGPL5   Progbuffer1   3.33E-01  4.45E-09  1.30E-12
[Pin Mapping]   pulldown_ref   pullup_ref
A1   NC   GVDD
A10   GND   NC
A11   GND   XPADVDD
A12   GND   NC
A13   GND   XPADVDD
A14   NC   XCOREVDD
A15   GND   XPADVDD
A16   NC   NVDDB
A17   GND   NVDDB
A18   GND   NVDDB
A19   NC   NVDDB
A2   GND   NC
A20   GND   NVDDB
A21   GND   NC
A22   GND   NVDDC
A23   NC   NVDDC
A3   GND   GVDD
A4   GND   GVDD
A5   GND   GVDD
A6   NC   GVDD
A7   GND   NVDDA
A8   GND   NVDDA
A9   GND   NVDDA
AA1   GND   GVDD
AA10   GND   NVDDK
AA11   NC   NVDDK
AA12   GND   NVDDK
AA13   GND   NVDDK
AA14   GND   NVDDK
AA15   GND   NVDDK
AA16   GND   NVDDK
AA17   GND   NVDDK
AA18   GND   NVDDK
AA19   GND   NVDDK
AA2   GND   GVDD
AA20   GND   NVDDK
AA21   GND   NVDDK
AA22   NC   NVDDJ
AA23   GND   NVDDJ
AA3   GND   GVDD
AA4   GND   NC
AA5   GND   NVDDP
AA6   GND   NVDDP
AA7   GND   NVDDP
AA8   GND   NVDDP
AA9   GND   NVDDP
AB1   GND   NC
AB10   GND   NVDDK
AB11   GND   NVDDK
AB12   GND   NC
AB13   GND   NVDDK
AB14   GND   NVDDK
AB15   GND   NVDDK
AB16   NC   NVDDK
AB17   GND   NVDDK
AB18   GND   NVDDK
AB19   GND   NC
AB2   GND   GVDD
AB20   GND   NVDDK
AB21   GND   NVDDK
AB22   NC   NVDDK
AB23   NC   NVDDJ
AB3   GND   GVDD
AB4   GND   NVDDP
AB5   GND   NVDDP
AB6   GND   NC
AB7   GND   NVDDP
AB8   NC   NVDDP
AB9   GND   NVDDK
AC1   NC   GVDD
AC10   GND   NVDDK
AC11   GND   NVDDK
AC12   GND   NVDDK
AC13   NC   NVDDK
AC14   GND   NVDDK
AC15   GND   NVDDK
AC16   GND   NVDDK
AC17   GND   NVDDK
AC18   GND   NVDDK
AC19   GND   NVDDK
AC2   GND   NC
AC20   GND   NVDDK
AC21   GND   NVDDK
AC22   GND   NVDDK
AC23   GND   NC
AC3   GND   GVDD
AC4   NC   NVDDP
AC5   GND   NVDDP
AC6   GND   NVDDP
AC7   GND   NVDDP
AC8   GND   NVDDP
AC9   GND   NC
B1   GND   NC
B10   NC   NVDDA
B12   NC   XCOREVDD
B13   GND   XPADVDD
B14   GND   NC
B15   GND   NC
B17   GND   NVDDB
B18   GND   NVDDB
B19   GND   NC
B2   GND   GVDD
B20   GND   NVDDC
B21   GND   NVDDC
B22   NC   NVDDC
B23   GND   NC
B3   NC   GVDD
B4   GND   GVDD
B5   GND   GVDD
B6   GND   GVDD
B7   NC   NVDDA
B8   GND   NVDDA
B9   GND   NVDDA
C1   GND   GVDD
C10   GND   NVDDA
C11   GND   NC
C12   GND   XPADVDD
C13   NC   XCOREVDD
C14   GND   XPADVDD
C15   GND   XPADVDD
C16   GND   NC
C17   GND   NVDDB
C18   NC   NVDDB
C19   GND   NVDDB
C2   GND   GVDD
C20   GND   NVDDC
C21   GND   NVDDC
C22   GND   NVDDC
C23   GND   NVDDC
C3   GND   GVDD
C4   GND   NC
C5   GND   GVDD
C6   GND   GVDD
C7   NC   NVDDA
C8   GND   NVDDA
C9   GND   NVDDA
D1   NC   GVDD
D10   GND   NVDDA
D11   GND   NC
D12   GND   XPADVDD
D13   GND   NC
D14   GND   NC
D15   NC   XPADVDD
D17   GND   NVDDB
D18   GND   NVDDB
D19   GND   NC
D2   GND   GVDD
D20   GND   NVDDC
D21   GND   NVDDC
D22   GND   NVDDC
D23   NC   NVDDC
D3   GND   GVDD
D4   GND   GVDD
D5   GND   GVDD
D6   GND   NC
D7   GND   NVDDA
D8   GND   NVDDA
D9   NC   NVDDA
E1   GND   GVDD
E2   GND   GVDD
E20   NC   NVDDC
E21   GND   NVDDC
E22   GND   NVDDC
E23   GND   NVDDC
E3   GND   NC
E4   GND   GVDD
F1   NC   GVDD
F10   NC   XPADVDD
F11   GND   XPADVDD
F12   GND   NC
F13   GND   XPADVDD
F14   NC   XPADVDD
F15   GND   NC
F16   GND   NVDDB
F17   GND   NC
F18   GND   NVDDC
F2   GND   GVDD
F20   GND   NVDDC
F21   GND   NVDDC
F22   GND   NVDDC
F23   GND   NC
F3   GND   GVDD
F4   GND   GVDD
F6   NC   GVDD
F7   GND   GVDD
F8   GND   NC
F9   NC   NVDDA
G1   GND   GVDD
G10   GND   NC
G11   GND   NC
G12   NC   SDAVDD
G13   GND   NC
G14   GND   NC
G15   GND   NC
G16   GND   NC
G17   GND   NC
G18   NC   NVDDC
G2   GND   GVDD
G20   GND   NC
G21   GND   NVDDF
G22   NC   NVDDF
G23   GND   NVDDF
G3   GND   GVDD
G4   NC   GVDD
G6   GND   GVDD
G7   GND   NC
G8   GND   NC
G9   GND   NVDDA
H1   GND   GVDD
H10   NC   VDD
H11   GND   NC
H12   GND   NC
H13   GND   NC
H14   NC   VDD
H15   NC   VDD
H16   NC   VDD
H17   GND   NC
H18   GND   NVDDF
H2   GND   NC
H20   GND   NVDDF
H21   GND   NVDDF
H22   GND   NVDDF
H23   GND   NC
H3   GND   GVDD
H4   GND   GVDD
H6   GND   NC
H7   GND   NC
H8   NC   VDD
H9   NC   VDD
J1   NC   GVDD
J10   GND   NC
J11   GND   NC
J12   GND   NC
J13   GND   NC
J14   GND   NC
J15   GND   NC
J16   NC   VDD
J17   GND   NVDDF
J18   GND   NVDDF
J2   GND   GVDD
J20   GND   NVDDF
J21   GND   NVDDF
J22   NC   NVDDF
J23   GND   NVDDF
J3   GND   GVDD
J4   NC   GVDD
J6   GND   GVDD
J7   GND   NC
J8   NC   VDD
J9   GND   NC
K1   GND   GVDD
K10   GND   NC
K11   GND   NC
K12   GND   NC
K13   GND   NC
K14   GND   NC
K15   GND   NC
K16   NC   VDD
K17   NC   NVDDF
K18   GND   NVDDF
K2   GND   GVDD
K20   GND   NVDDF
K21   GND   NVDDF
K22   GND   NVDDF
K23   GND   NVDDF
K3   GND   GVDD
K4   GND   GVDD
K6   GND   GVDD
K7   NC   GVDD
K8   NC   VDD
K9   GND   NC
L1   GND   NC
L10   GND   NC
L11   GND   NC
L12   GND   NC
L13   GND   NC
L14   GND   NC
L15   GND   NC
L16   NC   VDD
L17   GND   NVDDG
L18   GND   NVDDG
L2   GND   GVDD
L20   GND   NC
L21   GND   NVDDG
L22   GND   NVDDG
L23   GND   NVDDG
L3   GND   GVDD
L4   GND   GVDD
L6   GND   GVDD
L7   GND   NC
L8   NC   VDD
L9   GND   NC
M1   GND   GVDD
M10   GND   NC
M11   GND   NC
M12   GND   NC
M13   GND   NC
M14   GND   NC
M15   GND   NC
M16   NC   VDD
M17   NC   NVDDG
M18   GND   NVDDG
M2   GND   GVDD
M20   GND   NVDDG
M21   GND   NVDDG
M22   GND   NVDDG
M23   GND   NVDDG
M3   GND   GVDD
M4   GND   NC
M6   GND   GVDD
M7   GND   GVDD
M8   NC   VDD
M9   GND   NC
N1   NC   GVDD
N10   GND   NC
N11   GND   NC
N12   GND   NC
N13   GND   NC
N14   GND   NC
N15   GND   NC
N16   NC   VDD
N17   GND   NVDDH
N18   GND   NVDDG
N2   GND   GVDD
N20   GND   NVDDG
N21   GND   NVDDG
N22   NC   NVDDG
N23   GND   NVDDG
N3   GND   GVDD
N4   GND   GVDD
N6   GND   GVDD
N7   NC   GVDD
N8   NC   VDD
N9   GND   NC
P1   GND   GVDD
P10   GND   NC
P11   GND   NC
P12   GND   NC
P13   GND   NC
P14   GND   NC
P15   GND   NC
P16   NC   VDD
P17   NC   NVDDH
P18   GND   NVDDH
P2   GND   GVDD
P20   GND   NVDDH
P21   GND   NVDDH
P22   GND   NVDDG
P23   GND   NVDDG
P3   GND   GVDD
P4   GND   GVDD
P6   GND   NC
P7   GND   NC
P8   NC   VDD
P9   GND   NC
R1   GND   GVDD
R10   GND   NC
R11   GND   NC
R12   GND   NC
R13   GND   NC
R14   GND   NC
R15   GND   NC
R16   NC   VDD
R17   GND   NVDDH
R18   GND   NVDDH
R2   GND   NC
R20   NC   NVDDH
R21   GND   NVDDH
R22   GND   NC
R23   GND   NVDDH
R3   GND   GVDD
R4   GND   GVDD
R6   NC   AVDD1
R7   GND   NC
R8   NC   VDD
R9   GND   NC
T1   NC   GVDD
T10   NC   VDD
T11   NC   VDD
T12   NC   VDD
T13   NC   VDD
T14   NC   VDD
T15   NC   VDD
T16   NC   VDD
T17   NC   NVDDH
T18   GND   NVDDH
T2   GND   GVDD
T20   GND   NVDDH
T21   GND   NVDDH
T22   GND   NVDDH
T23   NC   NVDDH
T3   GND   GVDD
T4   NC   GVDD
T6   GND   NC
T7   GND   NC
T8   NC   VDD
T9   NC   VDD
U1   GND   GVDD
U10   NC   NVDDK
U11   GND   NVDDK
U12   GND   NVDDK
U13   GND   NVDDK
U14   NC   NVDDK
U15   GND   NVDDK
U16   GND   NVDDK
U17   GND   NC
U18   GND   NVDDK
U2   GND   GVDD
U20   GND   NVDDH
U21   GND   NC
U22   GND   NVDDH
U23   GND   NVDDH
U3   GND   GVDD
U4   GND   GVDD
U6   GND   GVDD
U7   NC   GVDD
U8   GND   NC
U9   GND   NVDDP
V1   GND   GVDD
V10   NC   AVDD2
V11   GND   NC
V12   GND   NVDDK
V13   GND   NVDDK
V14   GND   NVDDK
V15   GND   NVDDK
V16   GND   NVDDK
V17   GND   NVDDK
V18   GND   NVDDK
V2   GND   NC
V20   GND   NVDDH
V21   GND   NVDDH
V22   GND   NVDDH
V23   GND   NVDDH
V3   GND   GVDD
V4   GND   GVDD
V6   GND   GVDD
V7   GND   NC
V8   GND   NVDDP
V9   GND   NC
W1   GND   GVDD
W2   GND   GVDD
W20   GND   NC
W21   GND   NVDDH
W22   NC   NVDDH
W23   GND   NVDDH
W3   GND   GVDD
W4   GND   GVDD
Y1   GND   GVDD
Y10   GND   NVDDK
Y11   GND   NVDDK
Y12   GND   NVDDK
Y13   GND   NVDDK
Y14   GND   NVDDK
Y15   GND   NC
Y16   GND   NVDDK
Y17   GND   NVDDK
Y18   NC   NVDDK
Y19   GND   NVDDK
Y2   GND   GVDD
Y20   GND   NVDDK
Y21   GND   NVDDH
Y22   GND   NVDDJ
Y23   NC   STBY_1V
Y3   NC   GVDD
Y4   GND   GVDD
Y5   NC   NVDDP
Y6   GND   NVDDP
Y7   GND   NVDDP
Y8   GND   NC
Y9   GND   NVDDK
|*   Model Selector   *
[Model Selector] Progbuffer1
sta_io_253   gpio, 3.3V, 25 Ohm
sta_io_402   gpio, 2.5V, 40 Ohm
sta_io_403   gpio, 3.3V, 40 Ohm
sta_iod_253   gpio, 3.3V, 25 Ohm, Open Drain
sta_iod_402   gpio, 2.5V, 40 Ohm, Open Drain
sta_iod_403   gpio, 3.3V, 40 Ohm, Open Drain
[Model Selector] Progbuffer2
ddr1_typdrv_io   ddr1 mode, 2.5V, 18 Ohm
ddr1_mindrv_io   ddr1 mode, 2.5V, 18 Ohm
ddr1_maxdrv_io   ddr1 mode, 2.5V, 18 Ohm
ddr2_typdrv_io   ddr2 mode, 1.8V, 18 Ohm
ddr2_mindrv_io   ddr2 mode, 1.8V, 18 Ohm
ddr2_maxdrv_io   ddr2 mode, 1.8V, 18 Ohm
ddr2_maxdrv_75_io   ddr2 mode, 1.8V, 18 Ohm, 75 Ohm Termination
ddr2_mindrv_75_io   ddr2 mode, 1.8V, 18 Ohm, 75 Ohm Termination
ddr2_typdrv_75_io   ddr2 mode, 1.8V, 18 Ohm, 75 Ohm Termination
ddr2_maxdrv_150_io  ddr2 mode, 1.8V, 18 Ohm, 150 Ohm Termination
ddr2_mindrv_150_io  ddr2 mode, 1.8V, 18 Ohm, 150 Ohm Termination
ddr2_typdrv_150_io  ddr2 mode, 1.8V, 18 Ohm, 150 Ohm Termination
[Model Selector] tx_select
sdg_ohsdr100_004p   PCI Express: level 1.5
sdg_ohsdr100_006p   PCI Express: level 2.0
| End [Component] MPC8308
| Models and submodels in the file (28): ddr1_maxdrv_io (I/O), ddr1_mindrv_io (I/O), ddr1_typdrv_io (I/O), ddr2_maxdrv_150_io (Input), ddr2_maxdrv_75_io (Input), ddr2_maxdrv_io (I/O), ddr2_mindrv_150_io (Input), ddr2_mindrv_75_io (Input), ddr2_mindrv_io (I/O), ddr2_typdrv_150_io (Input), ddr2_typdrv_75_io (Input), ddr2_typdrv_io (I/O), pad_ae (Output), pouv_out (3-state), ptrmr100_cm (Input), rx_pzctl (Input), sdg_ohsdr100_004p (3-state), sdg_ohsdr100_00 (3-state), sdg_ohsdr100_04 (3-state), sdg_ohsdr100_06 (3-state), sdg_ohsdr100_006p (3-state), sta_io_253 (I/O), sta_io_402 (I/O), sta_io_403 (I/O), sta_iod_253 (I/O_open_drain), sta_iod_402 (I/O_open_drain), sta_iod_403 (I/O_open_drain), tx_pzctl (Input)
